| TEXAS INSTRUMENTS INCORPORATED
| Standard Linear and Logic Group
| IBIS Model of SN74LV161284
| 19-Bit Bus Interface
| This file contains package information for the following:
|  TSSOP 48-pin (DGG) package as [Component] SN74LV161284_DGG
|  SSOP 48-pin (DL) package as [Component] SN74LV161284_DL
| This device can be powered at the following Vccs:
|  3.3 volt Vcc
| This file provides unique models under the [Model Selector] for each mode.
| For operation at a specific mode, select the appropriate model after each
| [Model Selector] keyword.
[IBIS Ver]   3.2
[Comment char]  |_char
[File Name]   sn74lv161284.ibs
[File Rev]   1.1 | C_die
[Date]   July 19, 2007
[Source]   Data created from TI-SPICE simulations at TI-SLL.
[Notes]   The following is an IBIS list for the SN74LV161284.
   Please contact sllibis@ti.com with questions and
   comments concerning SLL IBIS models.
   -FILE REV HISTORY
   -1.1 Release IBIS file on 12/05/08.
   -End point warning due to DC and AC data Mismatch
   -The warning typ/min/max values never become zero- due to
   presence of pullup-resistor.
   -Non-monotonic data due to PMOS transistor connected to
   VCC CABLE.
   -VCC CABLE was equal to 5V during measurement.
   -Measurement method of C_comp in IBIS and Ci/Cio in datasheet
   is not same.
   -Power Clamp data deleted from control input model as there
   is no power-clamp diode.
[Disclaimer] Property of Texas Instruments Incorporated.  Unauthorized
   reproduction and/or distribution is strictly prohibited.
   This product is protected under copyright law.
   Created  2007, (C) Copyright  2007, Texas Instruments
   Incorporated, All Rights Reserved
   UNLESS THERE IS A SIGNED, WRITTEN AGREEMENT TO THE
   CONTRARY, TEXAS INSTRUMENTS (TI) IS PROVIDING THE IBIS
   MODELS  AND WITHOUT ANY WARRANTY, EXPRESSED OR
   IMPLIED.  TI assumes no liability for:
   1) the accuracy of the IBIS models provided to your
   company;
   2) the proper functioning of these IBIS Models in your
   design or for any resulting applications; or
   3) infringement of patents, copyrights or intellectual
   property rights resulting from your use of these IBIS
   models.
   TI provides IBIS Models as a service to our customers.
   You and your company shall not distribute, sell or give
   these models to anyone else without prior written
   permission from TI.
   TI reserves the right to make changes to our products or
   to discontinue any semiconductor product or service
   without notice, and advises our customers to obtain the
   latest version of relevant information to verify, before
   placing orders, that the information being relied on is
   current.
   Please be aware that your receipt and use of the IBIS
   information provided shall serve as acceptance of these
   terms and conditions.  If you do not accept these terms,
   you should return or destroy the IBIS models and any
   other accompanying information immediately.
| Component SN74LV161284_DGG 48-PIN TSSOP
[Component]   SN74LV161284_DGG
[Manufacturer]   Texas Instruments, Inc.
[Package]
|   typ   min   max
R_pkg   6.200e-02   5.000e-02   7.800e-02
L_pkg   3.527e-09   3.128e-09   4.255e-09
C_pkg   5.300e-13   4.170e-13   6.850e-13
[Pin]   signal_name   model_name   R_pin   L_pin   C_pin
1   HD   LV161284_HD   5.000e-02   4.250e-09   6.710e-13
2   A9   LV161284_AIN   5.700e-02   3.956e-09   6.740e-13
3   A10   LV161284_AIN   7.100e-02   3.922e-09   6.190e-13
4   A11   LV161284_AIN   7.800e-02   3.841e-09   6.180e-13
5   A12   LV161284_AIN   5.600e-02   3.535e-09   5.550e-13
6   A13   LV161284_AIN   5.800e-02   3.464e-09   5.030e-13
7   VCC   POWER   6.000e-02   3.362e-09   4.980e-13
8   A1   LV161284_AIO   6.100e-02   3.293e-09   4.620e-13
9   A2   LV161284_AIO   6.300e-02   3.240e-09   4.550e-13
10   GND   GND   6.300e-02   3.175e-09   4.420e-13
11   A3   LV161284_AIO   6.400e-02   3.153e-09   4.290e-13
12   A4   LV161284_AIO   6.500e-02   3.128e-09   4.180e-13
13   A5   LV161284_AIO   6.500e-02   3.128e-09   4.180e-13
14   A6   LV161284_AIO   6.400e-02   3.154e-09   4.290e-13
15   GND   GND   6.300e-02   3.174e-09   4.420e-13
16   A7   LV161284_AIO   6.300e-02   3.241e-09   4.550e-13
17   A8   LV161284_AIO   6.100e-02   3.293e-09   4.620e-13
18   VCC   POWER   6.000e-02   3.362e-09   4.970e-13
19   PLIN   LV161284_PLIN   5.800e-02   3.464e-09   5.030e-13
20   A14   LV161284_AOUT   5.600e-02   3.537e-09   5.600e-13
21   A15   LV161284_AOUT   7.700e-02   3.839e-09   6.260e-13
22   A16   LV161284_AOUT   7.100e-02   3.917e-09   6.270e-13
23   A17   LV161284_AOUT   5.800e-02   3.955e-09   6.850e-13
24   HLOUT   LV161284_HLOUT   5.200e-02   4.255e-09   6.790e-13
25   HLIN   LV161284_HLIN   5.100e-02   4.254e-09   6.760e-13
26   C17   LV161284_CIN   5.800e-02   3.957e-09   6.790e-13
27   C16   LV161284_CIN   7.100e-02   3.920e-09   6.210e-13
28   C15   LV161284_CIN   7.800e-02   3.843e-09   6.220e-13
29   C14   LV161284_CIN   5.600e-02   3.539e-09   5.600e-13
30   PLOUT   LV161284_PLOUT   5.800e-02   3.466e-09   5.030e-13
31   VCC_CABLE  POWER   6.000e-02   3.363e-09   4.970e-13
32   B8   LV161284_BIO   6.100e-02   3.294e-09   4.620e-13
33   B7   LV161284_BIO   6.300e-02   3.241e-09   4.540e-13
34   GND   GND   6.300e-02   3.175e-09   4.410e-13
35   B6   LV161284_BIO   6.400e-02   3.153e-09   4.290e-13
36   B5   LV161284_BIO   6.500e-02   3.129e-09   4.170e-13
37   B4   LV161284_BIO   6.500e-02   3.129e-09   4.170e-13
38   B3   LV161284_BIO   6.400e-02   3.152e-09   4.290e-13
39   GND   GND   6.400e-02   3.176e-09   4.410e-13
40   B2   LV161284_BIO   6.300e-02   3.241e-09   4.540e-13
41   B1   LV161284_BIO   6.100e-02   3.293e-09   4.620e-13
42   VCC_CABLE  POWER   6.000e-02   3.363e-09   4.970e-13
43   Y13   LV161284_YOUT   5.800e-02   3.464e-09   5.030e-13
44   Y12   LV161284_YOUT   5.600e-02   3.534e-09   5.610e-13
45   Y11   LV161284_YOUT   7.800e-02   3.841e-09   6.260e-13
46   Y10   LV161284_YOUT   7.100e-02   3.920e-09   6.220e-13
47   Y9   LV161284_YOUT   5.700e-02   3.955e-09   6.770e-13
48   DIR   LV161284_DIR   5.100e-02   4.252e-09   6.720e-13
| Component SN74LV161284_DL 48-PIN SSOP
[Component]   SN74LV161284_DL
[Manufacturer]   Texas Instruments, Inc.
[Package]
|   typ   min   max
R_pkg   4.800e-02   3.800e-02   5.300e-02
L_pkg   6.046e-09   5.084e-09   7.968e-09
C_pkg   8.130e-13   5.690e-13   1.157e-12
[Pin]   signal_name   model_name   R_pin   L_pin   C_pin
1   HD   LV161284_HD   4.600e-02   7.968e-09   1.017e-12
2   A9   LV161284_AIN   4.400e-02   7.299e-09   1.157e-12
3   A10   LV161284_AIN   4.300e-02   6.765e-09   1.058e-12
4   A11   LV161284_AIN   4.100e-02   6.269e-09   9.330e-13
5   A12   LV161284_AIN   3.800e-02   5.856e-09   8.290e-13
6   A13   LV161284_AIN   4.600e-02   5.802e-09   7.900e-13
7   VCC   POWER   5.000e-02   5.656e-09   7.380e-13
8   A1   LV161284_AIO   5.300e-02   5.500e-09   6.430e-13
9   A2   LV161284_AIO   5.200e-02   5.304e-09   6.060e-13
10   GND   GND   5.300e-02   5.189e-09   5.830e-13
11   A3   LV161284_AIO   5.100e-02   5.084e-09   5.690e-13
12   A4   LV161284_AIO   5.300e-02   5.862e-09   8.330e-13
13   A5   LV161284_AIO   5.300e-02   5.862e-09   8.330e-13
14   A6   LV161284_AIO   5.100e-02   5.084e-09   5.690e-13
15   GND   GND   5.300e-02   5.189e-09   5.830e-13
16   A7   LV161284_AIO   5.200e-02   5.304e-09   6.060e-13
17   A8   LV161284_AIO   5.300e-02   5.500e-09   6.430e-13
18   VCC   POWER   5.000e-02   5.656e-09   7.380e-13
19   PLIN   LV161284_PLIN   4.600e-02   5.802e-09   7.900e-13
20   A14   LV161284_AOUT   3.800e-02   5.856e-09   8.290e-13
21   A15   LV161284_AOUT   4.100e-02   6.269e-09   9.330e-13
22   A16   LV161284_AOUT   4.300e-02   6.765e-09   1.058e-12
23   A17   LV161284_AOUT   4.400e-02   7.299e-09   1.157e-12
24   HLOUT   LV161284_HLOUT   4.600e-02   7.968e-09   1.017e-12
25   HLIN   LV161284_HLIN   4.600e-02   7.968e-09   1.017e-12
26   C17   LV161284_CIN   4.400e-02   7.299e-09   1.157e-12
27   C16   LV161284_CIN   4.300e-02   6.765e-09   1.058e-12
28   C15   LV161284_CIN   4.100e-02   6.269e-09   9.330e-13
29   C14   LV161284_CIN   3.800e-02   5.856e-09   8.290e-13
30   PLOUT   LV161284_PLOUT   4.600e-02   5.802e-09   7.900e-13
31   VCC_CABLE  POWER   5.000e-02   5.656e-09   7.380e-13
32   B8   LV161284_BIO   5.300e-02   5.500e-09   6.430e-13
33   B7   LV161284_BIO   5.200e-02   5.304e-09   6.060e-13
34   GND   GND   5.300e-02   5.189e-09   5.830e-13
35   B6   LV161284_BIO   5.100e-02   5.084e-09   5.690e-13
36   B5   LV161284_BIO   5.300e-02   5.862e-09   8.330e-13
37   B4   LV161284_BIO   5.300e-02   5.862e-09   8.330e-13
38   B3   LV161284_BIO   5.100e-02   5.084e-09   5.690e-13
39   GND   GND   5.300e-02   5.189e-09   5.830e-13
40   B2   LV161284_BIO   5.200e-02   5.304e-09   6.060e-13
41   B1   LV161284_BIO   5.300e-02   5.500e-09   6.430e-13
42   VCC_CABLE  POWER   5.000e-02   5.656e-09   7.380e-13
43   Y13   LV161284_YOUT   4.600e-02   5.802e-09   7.900e-13
44   Y12   LV161284_YOUT   3.800e-02   5.856e-09   8.290e-13
45   Y11   LV161284_YOUT   4.100e-02   6.269e-09   9.330e-13
46   Y10   LV161284_YOUT   4.300e-02   6.765e-09   1.058e-12
47   Y9   LV161284_YOUT   4.400e-02   7.299e-09   1.157e-12
48   DIR   LV161284_DIR   4.600e-02   7.967e-09   1.017e-12
| Model LV161284_BIO
[Model Selector]   LV161284_BIO
LV161284_BIO_OD   Open-Drain Mode
LV161284_BIO_TP   Totem-Pole Mode
| Model LV161284_YOUT
[Model Selector]   LV161284_YOUT
LV161284_YOUT_OD   Open-Drain Mode
LV161284_YOUT_TP   Totem-Pole Mode
| Model LV161284_PLOUT
[Model Selector]   LV161284_PLOUT
LV161284_PLOUT_OD   Open-Drain Mode
LV161284_PLOUT_TP   Totem-Pole Mode
| Models and submodels in the file (15): LV161284_DIR (Input), LV161284_PLIN (Input), LV161284_AIN (Input), LV161284_HD (Input), LV161284_HLIN (Input), LV161284_CIN (Input), LV161284_AIO (I/O), LV161284_BIO_OD (I/O_open_drain), LV161284_AOUT (Output), LV161284_HLOUT (Output), LV161284_YOUT_OD (Open_drain), LV161284_PLOUT_OD (Open_drain), LV161284_PLOUT_TP (Output), LV161284_YOUT_TP (Output), LV161284_BIO_TP (I/O)
